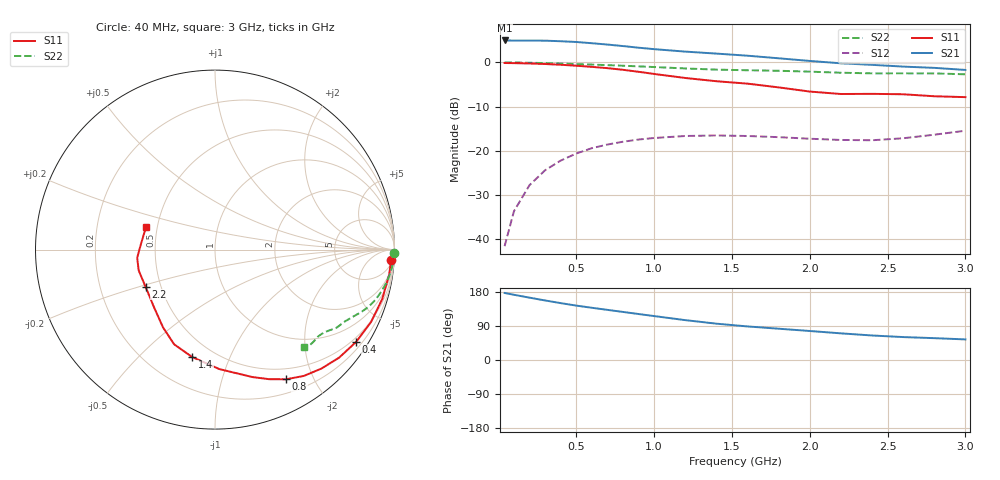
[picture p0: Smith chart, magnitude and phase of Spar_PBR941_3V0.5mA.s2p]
! Filename:  PBR941A.S2P  Version:  3.0
! NXP part #:  PBR941  Date: July 1998
! Bias condition:  Vce=3V, Ic=0.5mA
#  MHz  S  MA  R 50
! Freq  S11  S21  S12  S22
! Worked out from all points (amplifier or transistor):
!   21 points, 40 MHz to 3 GHz, reference 50 ohm
!   highest |S21| = 5.0 dB at 40 MHz (marker M1)
!   |S21| within 3 dB of that: start of sweep to 1.413 GHz
!   unconditionally stable (mu >= 1): 2.031 GHz to end of sweep
!   at 300 MHz: K = 0.14, MSG = 14.6 dB, |S12| = -24.4 dB
!   at 1 GHz: K = 0.42, MSG = 10.0 dB, |S12| = -17.1 dB
!   at 3 GHz: K = 1.18, MAG = 4.3 dB, |S12| = -15.5 dB
!   S11 on the Smith chart (normalised r, x): 40 MHz: 10, -32; 400 MHz: 0.38, -3.32; 800 MHz: 0.36, -1.63; 1.4 GHz: 0.38, -0.74; 2.2 GHz: 0.41, -0.21; 3 GHz: 0.43, +0.13
40  0.9833 -3.3  1.769 176.8  0.008365 87.1  0.9986 -1.2
100  0.9804 -8.1  1.763 172.1  0.02076 84.6  0.9966 -3.0
200  0.9718 -16.4  1.763 164.5  0.04095 79.6  0.9904 -5.9
300  0.9585 -24.8  1.759 157.1  0.06036 75.2  0.9812 -8.7
400  0.9397 -33.1  1.733 150.1  0.07757 70.5  0.9697 -11.4
500  0.9169 -41.0  1.7 143.6  0.09321 66.7  0.9569 -14.0
600  0.8894 -48.2  1.646 137.8  0.1071 62.7  0.9437 -16.2
700  0.8606 -54.9  1.59 132.3  0.1178 59.5  0.9305 -18.2
800  0.8243 -61.2  1.529 126.9  0.1267 56.4  0.9162 -20.0
900  0.7827 -67.3  1.465 121.3  0.1342 53.8  0.9013 -21.6
1000  0.7399 -73.7  1.411 116.0  0.1397 51.0  0.8857 -23.1
1200  0.6662 -87.9  1.323 105.2  0.1472 46.4  0.8537 -26.0
1400  0.6122 -101.9  1.257 95.9  0.1492 43.0  0.828 -28.8
1600  0.5749 -113.3  1.19 88.6  0.1472 42.3  0.8144 -31.1
1800  0.5216 -123.7  1.112 82.6  0.1428 43.7  0.8036 -32.9
2000  0.4679 -136.5  1.038 76.6  0.137 46.1  0.7853 -34.7
2200  0.4389 -151.9  0.976 70.3  0.1328 50.3  0.7637 -37.0
2400  0.4407 -164.7  0.9377 64.7  0.1317 56.8  0.7511 -40.0
2600  0.436 -174.0  0.8959 60.5  0.1387 64.9  0.7515 -43.1
2800  0.414 175.8  0.8668 57.6  0.1522 72.3  0.75 -45.4
3000  0.4045 161.7  0.8213 54.3  0.1688 78.3  0.7333 -47.4
